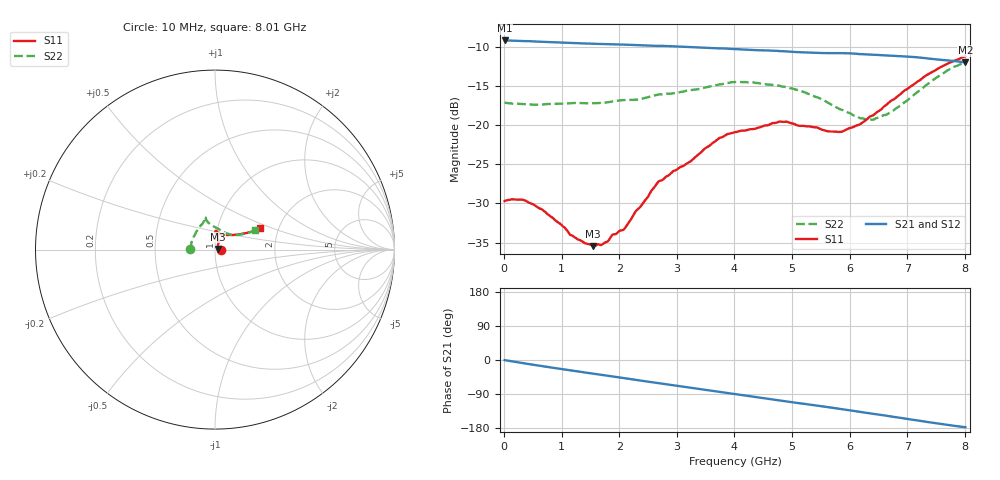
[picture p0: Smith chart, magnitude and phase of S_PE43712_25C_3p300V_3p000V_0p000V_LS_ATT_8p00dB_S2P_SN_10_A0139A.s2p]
! DEVICE ID: PE43712
! File Path: z:\PE43713\PE43713_CHAR_NOM_04292014\AMB\3p300\LS_ATT_8p00dB\PE43713_AMB_3p300V_3p000V_0p000V_LS_ATT_8p00dB_S2P_SN_10_A0139A.s2p
! Serial: 10
! Lot: A0139A
! Temp: 25C
! VDD: 3.300
! VSS: 0.000
! Control_Hi: 3.000
! Control_Lo: 0.000
! Attenuation Step: 8.00dB
! Port 1: RF1
! Port 2: RF2
! ThroughPath:1-2
! IDD: 0.0001466299
! ISS: -6.23e-008
#  Hz  S  RI  R  50
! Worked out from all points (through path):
!   801 points, 10 MHz to 8.01 GHz, reference 50 ohm
!   highest |S21| = -9.15 dB at 10 MHz (marker M1); lowest = -11.9 dB at 8.01 GHz (marker M2)
!   group delay of S21, straight-line fit = 60.9 ps
!   lowest |S11| = -35.5 dB at 1.55 GHz (marker M3), VSWR 1.03, Z = 51.7 + j0.386 ohm
!   |S11| at or under -10 dB: start of sweep to end of sweep
!   |S22| runs from -19.3 to -12.1 dB; largest |S21 - S12| = 0.0012
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1e7  0.0328 0.00013  0.3486 -0.0019  0.3487 -0.00187  -0.1395 0.000912
3e8  0.0332 -0.00392  0.3431 -0.0456  0.3431 -0.0456  -0.1359 0.0147
5e8  0.0308 -0.00534  0.3359 -0.0738  0.336 -0.0737  -0.1335 0.0235
9.6e8  0.0233 -0.00416  0.3113 -0.1323  0.3115 -0.1323  -0.1294 0.0458
1.17e9  0.0197 -0.00188  0.2972 -0.1558  0.2973 -0.156  -0.1265 0.0562
1.35e9  0.0181 0.000104  0.2844 -0.1752  0.2844 -0.1753  -0.1228 0.0638
1.55e9  0.0164 0.00374  0.2685 -0.1955  0.2686 -0.1955  -0.1166 0.0743
1.72e9  0.0157 0.00749  0.2542 -0.2117  0.2542 -0.2117  -0.1122 0.0823
2.09e9  0.0146 0.0161  0.2195 -0.2435  0.2196 -0.2434  -0.1038 0.1009
2.68e9  0.0201 0.0387  0.1563 -0.2813  0.1562 -0.2813  -0.0778 0.137
3.24e9  0.0164 0.0565  0.0903 -0.3033  0.0904 -0.3033  -0.0641 0.1547
3.72e9  0.0143 0.0806  0.0333 -0.3087  0.0331 -0.3086  -0.0571 0.1725
4.01e9  0.0105 0.0897  -0.000919 -0.3073  -0.000962 -0.3072  -0.0585 0.1797
4.79e9  0.0046 0.1056  -0.0865 -0.2854  -0.0866 -0.2856  -0.0512 0.1711
5.35e9  0.0151 0.0963  -0.1398 -0.2559  -0.1398 -0.2558  -0.0384 0.1509
5.63e9  0.0262 0.0875  -0.1637 -0.2391  -0.1636 -0.2391  -0.0194 0.1376
5.87e9  0.038 0.0828  -0.1853 -0.2219  -0.1851 -0.2219  0.000539 0.1254
6.31e9  0.0744 0.0811  -0.2165 -0.1835  -0.216 -0.1835  0.0455 0.0989
6.68e9  0.1124 0.0827  -0.2367 -0.1474  -0.2363 -0.1476  0.0857 0.0833
7.36e9  0.1883 0.0967  -0.2566 -0.0749  -0.2564 -0.0749  0.1614 0.0882
7.72e9  0.225 0.108  -0.2565 -0.0378  -0.2564 -0.038  0.2032 0.1002
8.01e9  0.2488 0.1208  -0.2524 -0.0114  -0.2522 -0.0118  0.2247 0.1078
